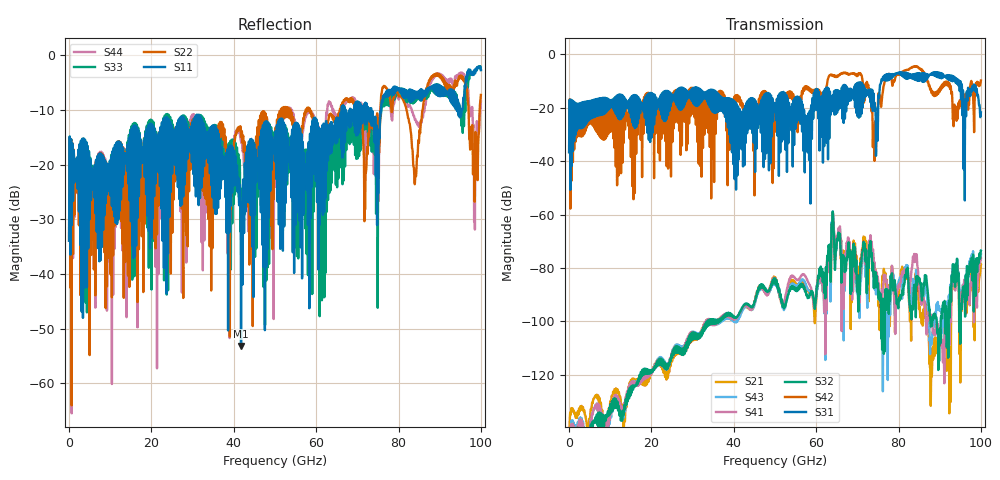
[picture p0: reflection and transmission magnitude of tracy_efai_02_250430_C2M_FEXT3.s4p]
!! PART DESCRIPTION: TE 224G+ VSR Channel- Chip to module, IO connector to CPC(Co-packaged connector) through over the board cable
!! CHANNEL DESCRIPTION: Module trace -> Mated IO 224G+ Connector -> Internal Cable Termination -> 30AWG 300mm Cable -> Cable
!!  termination + CPC connector(No footprint or package included)
!! MODEL REVISION:  Rev 3, Created on April 25, 2025
!! MODEL STATUS: Development
!! MODEL GEOMETRY: 8 Pair Channel
!! MODEL FREQUENCY RANGE: 0 GHz to 100 GHz in 10.00 MHz frequency steps
!! MODEL EDGE RATE LIMITATION: 5ps (Using conservative 0.5/Fmax rule of thumb)
!! PORT DEFINITIONS:
!! Port  1  ----->  Module Side  -->  Host Side, A Row  <-----  Port  2
!! Port  3  ----->  Module Side  -->  Host Side, A Row  <-----  Port  4
# GHz S MA R 45
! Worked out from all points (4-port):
!   10000 points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, 10 MHz to 100 GHz, reference 45 ohm
!   strongest paths, dB at 10 MHz, 25.01 GHz, 50.01 GHz, 75.01 GHz, 100 GHz:
!     S31: -36.7, -17.7, -20.3, -22.6, -21.7
!     S42: -36.6, -18.4, -28.2, -17.6, -9.8
!     S32: -150.9, -113.5, -84.1, -86.7, -73.4
!     S41: -151.1, -113.4, -84.0, -84.0, -76.2
!     S43: -150.7, -113.1, -84.9, -85.2, -74.6
!     S21: -148.6, -115.0, -83.6, -87.7, -78.5
!   lowest |S11| = -53.2 dB at 41.76 GHz (marker M1), VSWR 1.00, Z = 44.9 + j0.179 ohm
!   |S11| at or under -10 dB: start of sweep to 66.19 GHz; 67.15 GHz to 68.21 GHz (1.059 GHz wide, 1.57 % of centre); 73.39 GHz to 75.75 GHz (2.363 GHz wide, 3.17 % of centre)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
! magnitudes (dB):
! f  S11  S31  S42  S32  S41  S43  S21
! 10 MHz  -33.9  -36.7  -36.6  -150.9  -151.1  -150.7  -148.6
! 41.76 GHz  -53.2  -22.0  -17.2  -95.6  -95.7  -96.9  -96.1
! 44.18 GHz  -23.2  -26.5  -23.6  -94.7  -95.6  -95.6  -95.7
! 70.53 GHz  -8.8  -10.5  -7.4  -89.3  -93.1  -98.7  -85.3
! 74.21 GHz  -16.0  -19.1  -32.3  -86.5  -81.7  -84.4  -83.4
! 77.52 GHz  -7.2  -7.4  -7.6  -91.4  -89.4  -102.5  -89.9
! 100 GHz  -2.7  -21.7  -9.8  -73.4  -76.2  -74.6  -78.5
